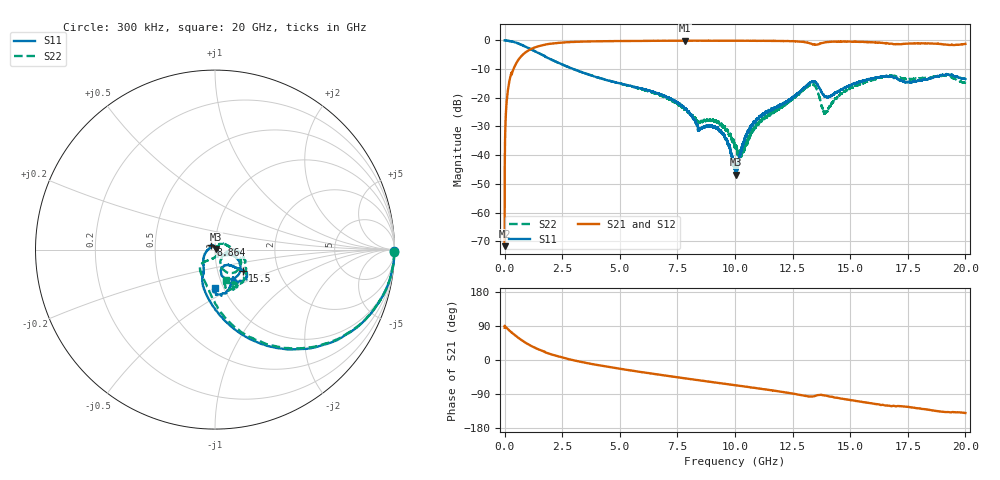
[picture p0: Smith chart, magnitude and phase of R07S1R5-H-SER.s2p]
!{R07S1R5}
!Johanson Technology Inc.
!www.johansontechnology.com
!Test Board Conditions:
!Substrate Type  RO4350B
!Substrate Thickness  10 mil
!Substrate Dk  3.66
!TL Type: GCPW
!TL Trace Width  21 mil
!TL Gap  20 mil
!Electrode orientation  Horizontal
!DUT TOPOLOGY	SERIES
!Mounting Pad LxW  16x21 mil
! Created Sat Feb  6 11:19:45 2021
# hz S ma R 50
! 2 Port Network Data from SP1.SP block
! freq  magS11  angS11  magS21  angS21  magS12  angS12  magS22  angS22
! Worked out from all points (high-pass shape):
!   20001 points, 300 kHz to 20 GHz, reference 50 ohm
!   highest |S21| = -0.07 dB at 7.844 GHz (marker M1); lowest = -71.7 dB at 300 kHz (marker M2)
!   |S21| within 3 dB of the highest: 1.131 GHz to end of sweep
!   lowest |S11| = -46.8 dB at 10.04 GHz (marker M3), VSWR 1.01, Z = 50.3 + j0.324 ohm
!   |S11| at or under -10 dB: 2.987 GHz to end of sweep
!   |S22| runs from -40.9 to 0.0 dB; largest |S21 - S12| = 0.012
!   S11 on the Smith chart (normalised r, x): 300 kHz: open; 8.864 GHz: 0.95, +0.05; 15.5 GHz: 1.32, -0.32; 20 GHz: 0.91, -0.41
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300000  0.9996 -0.5  0.0002588 85.1  0.0003547 114.0  1 -0.6
1.013e8  0.9936 -6.3  0.09676 84.0  0.09696 84.0  0.994 -6.2
1.323e8  0.9916 -8.2  0.1263 82.0  0.1262 82.1  0.991 -8.2
2.563e8  0.969 -15.7  0.2389 74.9  0.2385 74.8  0.969 -15.5
4.993e8  0.9145 -26.7  0.3969 63.1  0.3963 63.1  0.9154 -26.3
1.0343e9  0.7368 -48.7  0.6698 41.3  0.6694 41.3  0.7381 -48.0
1.8503e9  0.5024 -71.8  0.8597 18.4  0.8595 18.5  0.5001 -70.5
3.3343e9  0.281 -96.8  0.955 -5.2  0.9546 -5.2  0.2819 -91.8
6.6673e9  0.1199 -122.3  0.9868 -38.3  0.9869 -38.4  0.1147 -133.1
7.8443e9  0.06468 -154.2  0.9917 -48.5  0.9895 -48.6  0.06266 -117.0
8.4673e9  0.02777 149.8  0.9902 -53.7  0.9905 -53.8  0.03661 -77.8
8.8643e9  0.03335 133.1  0.9909 -57.1  0.9898 -57.1  0.04097 -68.8
9.5523e9  0.02088 118.3  0.9894 -62.8  0.9894 -62.8  0.03167 -61.3
1.00003e10  0.005856 63.0  0.9899 -66.5  0.989 -66.6  0.01346 -39.3
1.00363e10  0.004579 44.7  0.9881 -66.8  0.9888 -66.9  0.01498 -41.1
1.03193e10  0.01468 -28.1  0.9875 -69.1  0.988 -69.1  0.01138 16.2
1.08803e10  0.03788 -38.2  0.9861 -73.9  0.9841 -73.8  0.03072 57.2
1.33343e10  0.1914 -46.4  0.8701 -96.4  0.8704 -96.4  0.1712 -38.6
1.39313e10  0.1059 -66.3  0.9317 -93.9  0.9307 -93.9  0.05552 -32.4
1.54963e10  0.1945 -37.4  0.9486 -110.3  0.9435 -110.2  0.1798 -20.0
1.66673e10  0.232 -46.0  0.876 -120.3  0.8794 -120.8  0.2429 -52.9
2e10  0.2123 -90.2  0.8699 -139.9  0.8648 -139.8  0.1823 -70.0
